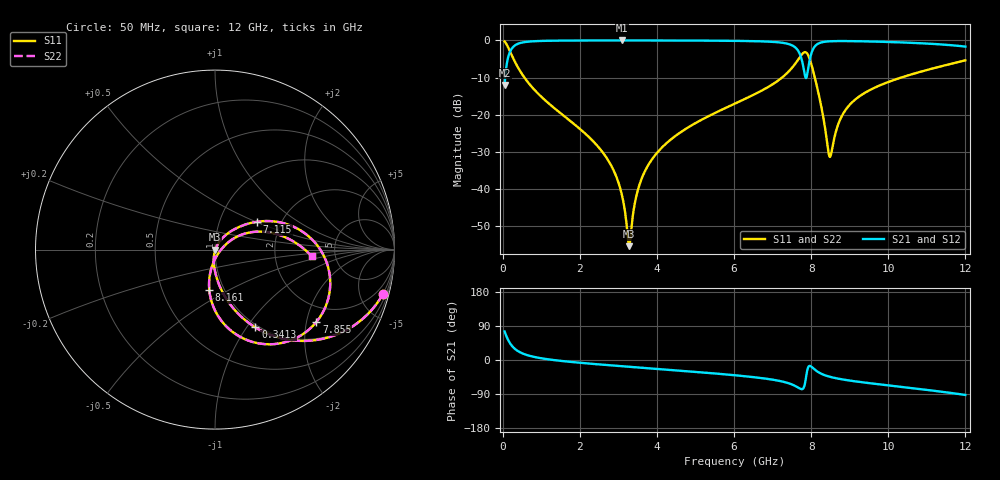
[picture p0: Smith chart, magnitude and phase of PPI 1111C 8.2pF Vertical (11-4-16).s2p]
# GHz S MA R 50
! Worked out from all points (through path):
!   1601 points, 50 MHz to 12 GHz, reference 50 ohm
!   highest |S21| = -0.02 dB at 3.082 GHz (marker M1); lowest = -12.0 dB at 50 MHz (marker M2)
!   group delay of S21, straight-line fit = 23.3 ps
!   lowest |S11| = -55.3 dB at 3.284 GHz (marker M3), VSWR 1.00, Z = 50.2 - j0.041 ohm
!   |S11| at or under -10 dB: 563.8 MHz to 7.244 GHz (6.681 GHz wide, 171 % of centre); 8.095 GHz to 10.33 GHz (2.237 GHz wide, 24.3 % of centre)
!   |S22| runs from -55.3 to -0.3 dB; largest |S21 - S12| = 0
!   S11 on the Smith chart (normalised r, x): 50 MHz: 0.96, -7.57; 341.3 MHz: 0.97, -1.10; 7.115 GHz: 1.51, +0.51; 7.855 GHz: 1.47, -2.29; 8.161 GHz: 0.85, -0.40; 12 GHz: 3.30, -0.34
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0.05  0.9679 -14.8  0.2512 75.2  0.2512 75.2  0.9679 -14.8
0.1769688  0.7356 -43.6  0.6771 46.4  0.6771 46.4  0.7356 -43.6
0.3412812  0.4882 -62.6  0.8722 27.3  0.8722 27.3  0.4882 -62.6
0.7894062  0.2263 -81.1  0.9732 8.7  0.9732 8.7  0.2263 -81.1
2.044156  0.06181 -96.5  0.9967 -7.7  0.9967 -7.7  0.06181 -96.5
2.723813  0.02497 -100.0  0.998 -13.5  0.998 -13.5  0.02497 -100.0
3.082313  0.008775 -95.6  0.9981 -16.3  0.9981 -16.3  0.008775 -95.6
3.283969  0.00171 -13.8  0.9981 -17.9  0.9981 -17.9  0.00171 -13.8
3.560313  0.01201 61.3  0.9979 -20.1  0.9979 -20.1  0.01201 61.3
4.038312  0.03229 62.7  0.9973 -23.8  0.9973 -23.8  0.03229 62.7
6.025  0.1415 48.2  0.9859 -40.3  0.9859 -40.3  0.1415 48.2
7.115437  0.2816 33.5  0.9462 -53.9  0.9462 -53.9  0.2816 33.5
7.608375  0.5027 11.0  0.7865 -69.7  0.7865 -69.7  0.5027 11.0
7.765219  0.6535 -12.3  0.5266 -76.9  0.5266 -76.9  0.6535 -12.3
7.854844  0.6941 -35.5  0.3162 -53.5  0.3162 -53.5  0.6941 -35.5
8.019156  0.4499 -79.9  0.702 -18.7  0.702 -18.7  0.4499 -79.9
8.161062  0.2269 -98.1  0.8909 -30.5  0.8909 -30.5  0.2269 -98.1
8.489688  0.02712 -32.3  0.973 -44.4  0.973 -44.4  0.02712 -32.3
8.721219  0.07918 28.0  0.9796 -49.6  0.9796 -49.6  0.07918 28.0
8.95275  0.1276 30.7  0.9787 -53.6  0.9787 -53.6  0.1276 30.7
10.01331  0.2772 21.2  0.9521 -67.1  0.9521 -67.1  0.2772 21.2
12  0.5396 -3.9  0.8253 -92.2  0.8253 -92.2  0.5396 -3.9
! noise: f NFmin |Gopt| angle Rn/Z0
0.05  0.0004033  0.8829  2.101  0.0007467
1.372  0.003797  0.6776  8.07  0.002264
2.701  0.006293  0.6312  14.93  0.003154
4.031  0.008736  0.6144  21.64  0.004071
5.36  0.0118  0.6265  28.15  0.005586
6.682  0.01965  0.7138  34.72  0.01238
8.012  0.1491  0.9502  41.91  0.586
9.341  0.02754  0.7309  47.48  0.01717
10.67  0.02807  0.714  52.65  0.01567
12  0.04193  0.7855  58.43  0.03075
